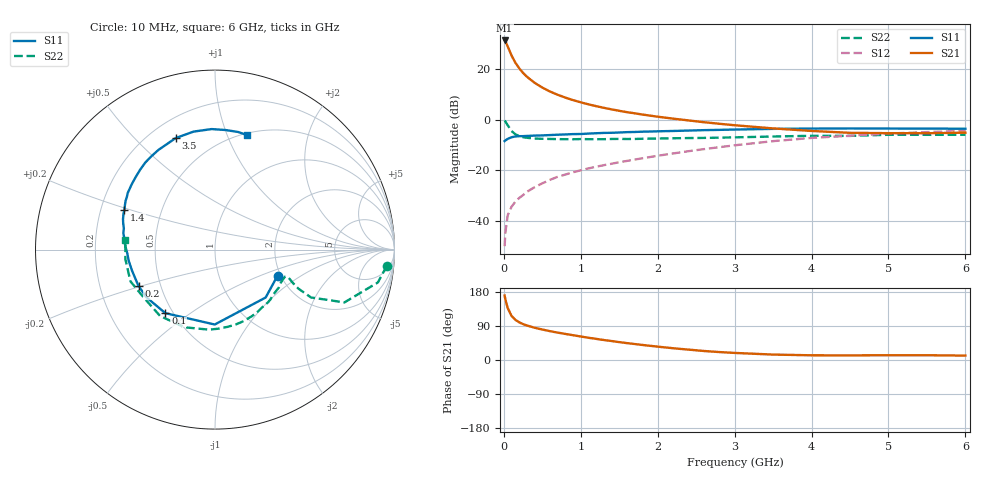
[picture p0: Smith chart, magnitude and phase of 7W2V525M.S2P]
! Infineon Technologies  Discrete & RF Semiconductors
! BFS17W
! Si NPN RF Bipolar Junction Transistor in SOT323
! VCE = 2.5 V  IC = 25 mA
! Common Emitter S-Parameters:  August  1999
# GHz  S  MA  R  50
!  f  S11  S21  S12  S22
! GHz  MAG  ANG  MAG  ANG  MAG  ANG  MAG  ANG
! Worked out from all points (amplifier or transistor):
!   36 points, 10 MHz to 6 GHz, reference 50 ohm
!   highest |S21| = 31.5 dB at 10 MHz (marker M1)
!   |S21| within 3 dB of that: start of sweep to 59.19 MHz
!   unconditionally stable (mu >= 1): 217.5 MHz to 2.505 GHz; 4.163 GHz to end of sweep
!   at 250 MHz: K = 1.07, MAG = 22.6 dB, |S12| = -29.9 dB
!   at 1.4 GHz: K = 1.22, MAG = 8.0 dB, |S12| = -17.5 dB
!   at 6 GHz: K = 1.09, MAG = -2.1 dB, |S12| = -4.4 dB
!   S11 on the Smith chart (normalised r, x): 10 MHz: 1.93, -0.65; 100 MHz: 0.45, -0.40; 200 MHz: 0.37, -0.20; 1.4 GHz: 0.30, +0.19; 3.5 GHz: 0.30, +0.66; 6 GHz: 0.52, +1.18
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0.01  0.3776 -22.6  37.43 170.1  0.0031 83.1  0.9617 -5.4
0.02  0.3885 -43.4  35.93 160.1  0.0057 80.5  0.9258 -11.4
0.05  0.4174 -90.2  28.61 137.1  0.0127 65.3  0.7788 -22.2
0.1  0.4494 -128.0  18.85 116.5  0.0188 59.0  0.5979 -26.5
0.15  0.4658 -145.4  13.53 105.9  0.0237 60.1  0.5134 -25.1
0.2  0.4717 -154.6  10.48 99.5  0.0281 61.8  0.4743 -23.3
0.25  0.4728 -161.2  8.5 94.7  0.032 63.4  0.4504 -21.7
0.3  0.4771 -166.0  7.138 91.1  0.0372 65.3  0.439 -21.0
0.4  0.485 -172.7  5.409 85.1  0.0459 67.0  0.4233 -20.6
0.5  0.4887 -177.3  4.348 80.4  0.0547 69.1  0.4185 -21.1
0.6  0.4966 179.1  3.626 76.1  0.0642 70.0  0.4155 -22.3
0.7  0.5047 175.8  3.13 72.3  0.0738 70.7  0.4127 -24.0
0.9  0.519 169.7  2.45 65.4  0.0907 70.9  0.4098 -28.3
1.1  0.5317 164.1  2.021 58.7  0.1083 71.0  0.4114 -33.5
1.4  0.5509 156.4  1.606 50.1  0.1339 71.4  0.4154 -42.1
1.8  0.5797 147.0  1.27 39.7  0.1719 71.3  0.4192 -54.8
2.2  0.5986 137.7  1.052 31.0  0.2143 70.2  0.4289 -67.6
2.8  0.6296 124.1  0.832 21.0  0.2854 66.3  0.4412 -87.8
3.5  0.6588 109.4  0.673 14.3  0.376 59.2  0.4649 -111.4
4.5  0.6718 91.6  0.55 12.2  0.4817 45.7  0.4781 -145.5
5.5  0.6679 79.0  0.54 12.6  0.5683 33.1  0.502 -173.8
6  0.6627 74.2  0.554 11.6  0.6028 27.1  0.5025 173.8
